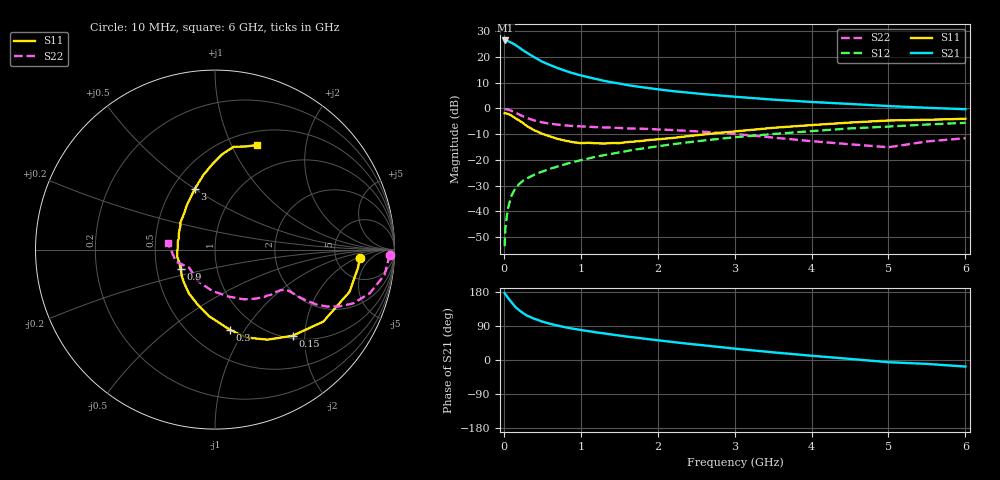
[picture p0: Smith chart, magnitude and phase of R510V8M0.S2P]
! SIEMENS Small Signal Semiconductors
! BFR183
! Si NPN RF Bipolar Junction Transistor in SOT23
! VCE = 10 V  IC = 8 mA
! Common Emitter S-Parameters:  May  1996
# GHz  S  MA  R  50
!  f  S11  S21  S12  S22
! GHz  MAG  ANG  MAG  ANG  MAG  ANG  MAG  ANG
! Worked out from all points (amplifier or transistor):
!   36 points, 10 MHz to 6 GHz, reference 50 ohm
!   highest |S21| = 26.4 dB at 20 MHz (marker M1)
!   |S21| within 3 dB of that: start of sweep to 210.5 MHz
!   unconditionally stable (mu >= 1): 894.1 MHz to 2.716 GHz
!   at 250 MHz: K = 0.53, MSG = 25.3 dB, |S12| = -28.1 dB
!   at 1.4 GHz: K = 1.05, MAG = 12.5 dB, |S12| = -17.7 dB
!   at 6 GHz: K = 0.88, MSG = 2.6 dB, |S12| = -5.6 dB
!   S11 on the Smith chart (normalised r, x): 10 MHz: 8.68, -2.46; 150 MHz: 1.05, -1.74; 300 MHz: 0.76, -0.86; 900 MHz: 0.67, -0.15; 3 GHz: 0.65, +0.50; 6 GHz: 0.65, +1.26
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0.01  0.8074 -3.5  20.72 176.6  0.0021 83.1  0.9769 -1.7
0.02  0.8035 -7.1  20.92 173.4  0.0047 81.8  0.9679 -3.4
0.05  0.7856 -17.4  20.47 165.1  0.0109 80.9  0.9548 -8.5
0.1  0.7246 -33.6  18.85 152.3  0.0202 73.0  0.8963 -15.7
0.15  0.6461 -48.0  17.14 140.0  0.0279 68.1  0.826 -21.3
0.2  0.5806 -59.8  15.2 131.2  0.0339 65.4  0.7582 -24.7
0.25  0.5203 -70.3  13.46 123.6  0.0394 62.0  0.7011 -26.9
0.3  0.4531 -79.6  12.04 117.3  0.0437 61.9  0.6513 -28.3
0.4  0.3731 -95.0  9.782 108.6  0.0518 61.0  0.5801 -29.2
0.5  0.3205 -107.7  8.081 101.3  0.0593 61.0  0.5354 -29.4
0.6  0.2849 -120.4  6.959 95.6  0.0669 61.4  0.5056 -29.3
0.7  0.2552 -131.9  6.09 90.7  0.0744 62.1  0.484 -29.2
0.9  0.22 -150.3  4.818 82.7  0.0904 62.8  0.455 -29.4
1.1  0.2143 -169.1  4.034 76.1  0.1067 62.8  0.44 -30.8
1.3  0.2072 175.5  3.448 70.2  0.1233 62.5  0.4267 -32.2
1.6  0.2208 155.6  2.856 61.8  0.1485 61.4  0.4093 -35.4
2.2  0.2668 129.8  2.166 47.4  0.2018 57.4  0.3793 -44.0
3  0.3563 108.4  1.688 30.0  0.275 49.6  0.3196 -60.1
3.5  0.4194 99.0  1.481 20.2  0.3175 43.8  0.2713 -74.2
4.5  0.5308 85.9  1.221 2.9  0.4082 32.3  0.2008 -117.9
5.5  0.6004 73.2  1.028 -10.3  0.4863 20.8  0.2278 -163.0
6  0.6287 68.0  0.965 -17.3  0.5248 13.2  0.2635 172.4
